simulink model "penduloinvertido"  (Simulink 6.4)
settings: Solver=ode45  SolverMode=SingleTasking  StartTime=0  StopTime=100  MaxStep=0.005  RelTol=1e-6  AbsTol=1e-6
libraries: simulink x1

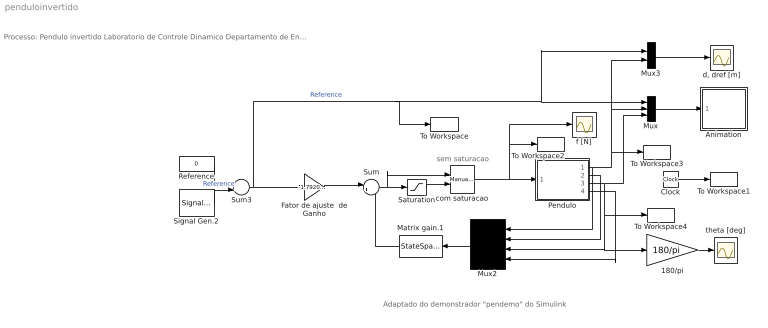
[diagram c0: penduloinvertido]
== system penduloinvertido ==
  note: Processo: Pendulo invertido Laboratorio de Controle Dinamico Departamento de Eng. Eletrica (ENE) Universidade de Brasilia (UnB)
  note: Adaptado do demonstrador "pendemo" do Simulink
  note: sem saturacao
  180/pi : Gain  Gain=180/pi
  Animation : Subsystem  mask(Pendulum plot){}
      mask help: Pendulum plot
      mask init:
      | RefBlock=&1;
  Clock : Clock
  Fator de ajuste  de Ganho : Gain  Gain=-1.79202901210101
  Matrix gain.1 : StateSpace  Orientation=left  A=[]  B=[]  C=[]  D=K  mask(Matrix gain){K=[-1.79202901210101  -2.86748729196427 -21.42671889993964  -3.37253362404895]}
      mask prompts: K "Gain matrix:"
      mask help: Matrix Gain:
  Mux : Mux  Inputs=3
  Mux2 : Mux  Orientation=left
  Mux3 : Mux  Inputs=2
  Pendulo : Subsystem  mask(Inverted pendulum on cart){}
      mask help: Unmask and double-click to see dynamics
      mask init:
      | M=@1; m=@2; l=@3; g=@4;
  Reference : Constant  Value=0  OutDataType=sfix(16)  ConRadixGroup=Use specified scaling  OutScaling=2^0  SampleTime=inf  FramePeriod=inf
  Saturation : Saturate  UpperLimit=3  LowerLimit=-3
  Signal Gen.2 : SignalGenerator  WaveForm=square  Amplitude=4  Frequency=0.024
  Sum : Sum  Inputs=|+-
  Sum3 : Sum
  To Workspace : ToWorkspace  VariableName=dref  SampleTime=0.1  SaveFormat=Array
  To Workspace1 : ToWorkspace  VariableName=t  SampleTime=0.1  SaveFormat=Array
  To Workspace2 : ToWorkspace  VariableName=f  SampleTime=0.1  SaveFormat=Array
  To Workspace3 : ToWorkspace  VariableName=d  SampleTime=0.1  SaveFormat=Array
  To Workspace4 : ToWorkspace  VariableName=theta  SampleTime=0.1  SaveFormat=Array
  com saturacao : simulink/Signal Routing/Manual Switch  SystemSampleTime=-1  sw=1  action=0
  "d, dref [m]" : Scope
  f [N] : Scope
  theta [deg] : Scope
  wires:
  Mux/1 -> Animation/1(in_1)
  Pendulo/3(theta) -> Mux/3, To Workspace4/1, Mux2/3, 180/pi/1
  Pendulo/1(d) -> Mux2/1, To Workspace3/1, Mux/2, Mux3/2
  Clock/1 -> To Workspace1/1
  Sum/1 -> Saturation/1, com saturacao/1
  Fator de ajuste  de Ganho/1 -> Sum/1
  Pendulo/2(d(d)/dt) -> Mux2/2
  Pendulo/4(d(theta)/dt) -> Mux2/4
  Sum3/1 -> To Workspace/1, Mux/1, Mux3/1, Fator de ajuste  de Ganho/1  "Reference"
  Mux3/1 -> "d, dref [m]"/1
  180/pi/1 -> theta [deg]/1
  Mux2/1 -> Matrix gain.1/1
  Matrix gain.1/1 -> Sum/2
  com saturacao/1 -> Pendulo/1(f), To Workspace2/1, f [N]/1
  Saturation/1 -> com saturacao/2
  Signal Gen.2/1 -> Sum3/2  "Reference"
  Reference/1 -> Sum3/1

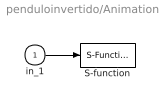
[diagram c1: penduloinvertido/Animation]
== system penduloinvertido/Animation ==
  in_1 : Inport
  S-function : S-Function  FunctionName=pendan  Parameters=RefBlock
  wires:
  in_1/1 -> S-function/1

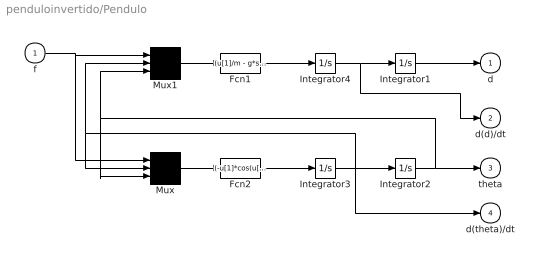
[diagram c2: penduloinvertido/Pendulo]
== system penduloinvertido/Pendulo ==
  f : Inport
  Fcn1 : Fcn  Expr=(u[1]/m - g*sin(u[3])*cos(u[3]) + l*power(u[2],2)*sin(u[3]))/(M/m + power(sin(u[3]),2))
  Fcn2 : Fcn  Expr=(-u[1]*cos(u[3])/m + (M+m)*g*sin(u[3])/m - l*power(u[2],2)*sin(u[3])*cos(u[3]))/(l*(M/m + power(sin(u[3]),2)))
  Integrator{1..4} (4 alike) : Integrator
  Mux : Mux  Inputs=3
  Mux1 : Mux  Inputs=3
  d : Outport  InitialOutput=0
  d(d)/dt : Outport  Port=2  InitialOutput=0
  theta : Outport  Port=3  InitialOutput=0
  d(theta)/dt : Outport  Port=4  InitialOutput=0
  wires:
  Integrator1/1 -> d/1
  Fcn2/1 -> Integrator3/1
  Mux/1 -> Fcn2/1
  Mux1/1 -> Fcn1/1
  Fcn1/1 -> Integrator4/1
  Integrator4/1 -> Integrator1/1, d(d)/dt/1
  f/1 -> Mux1/1, Mux/1
  Integrator3/1 -> Integrator2/1, Mux1/2, Mux/2, d(theta)/dt/1
  Integrator2/1 -> theta/1, Mux1/3, Mux/3
